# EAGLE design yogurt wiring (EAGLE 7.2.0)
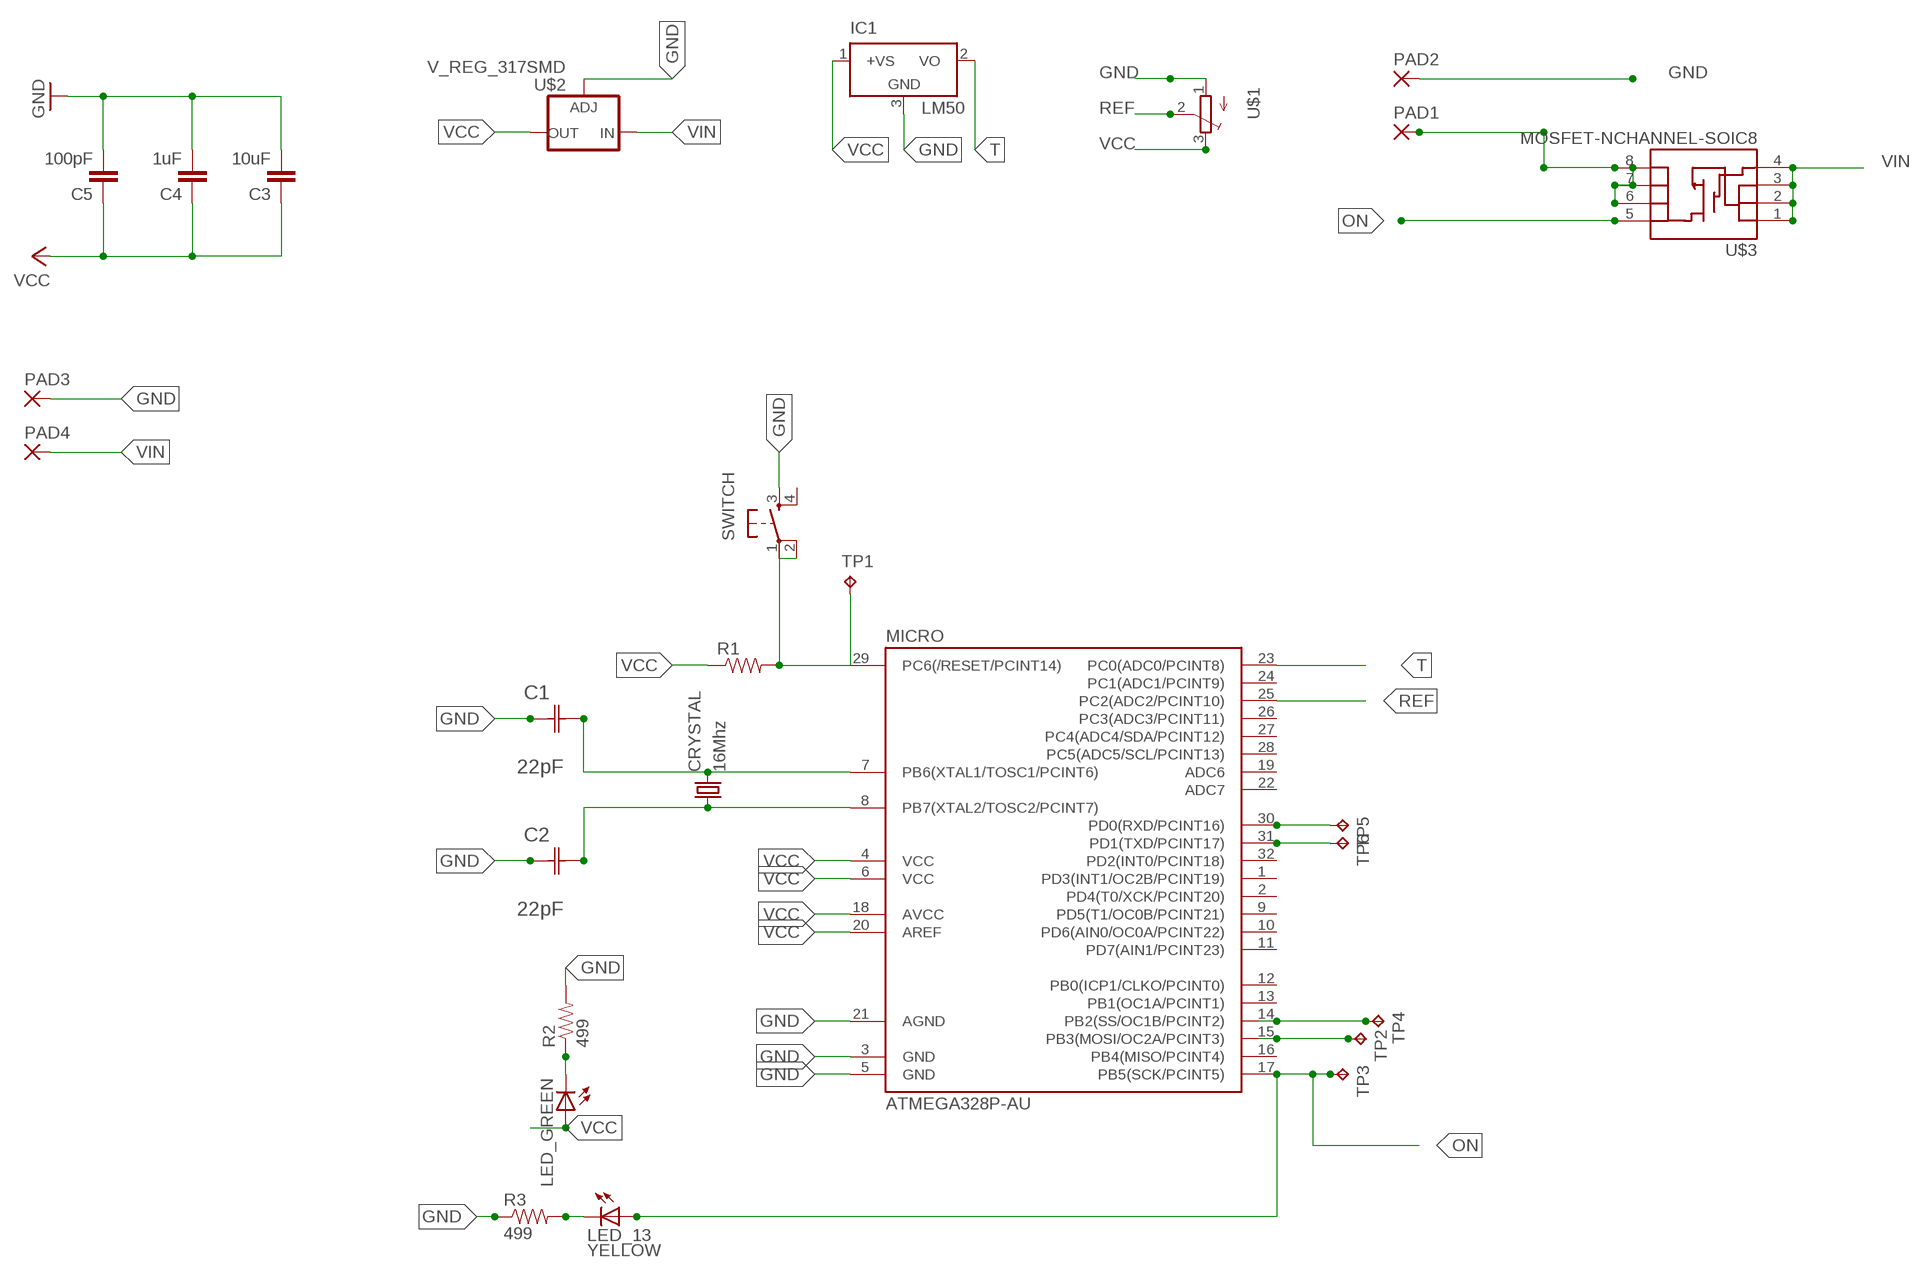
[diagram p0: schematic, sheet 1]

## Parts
C1  22pF  0612ZC225MAT2A  [CAPC3216X178N]
C2  22pF  0612ZC225MAT2A  [CAPC3216X178N]
C3  10uF  CAP1206  [1206]
C4  1uF  CAP1206  [1206]
C5  100pF  CAP1206  [1206]
CRYSTAL  16Mhz  CSM-7X-DU  [CSM-7X-DU]
IC1  LM50  [SOT23]
LED_13  YELLOW  LED1206  [1206]
LED_GREEN  LED1206  [1206]
MICRO  ATMEGA328P-AU  ATMEGA48/88/168-AU  [TQFP32-08]
PAD1  SMD5  [SMD2,54-5,08]
PAD2  SMD5  [SMD2,54-5,08]
PAD3  SMD5  [SMD2,54-5,08]
PAD4  SMD5  [SMD2,54-5,08]
R1  RESISTOR1206  [1206]
R2  499  RESISTOR1206  [1206]
R3  499  RESISTOR1206  [1206]
SWITCH  6MM_SWITCH6MM_SWITCH  [6MM_SWITCH]
TP1  TPPAD1-17Y  [P1-17Y]
TP2  TPPAD1-17Y  [P1-17Y]
TP3  TPPAD1-17Y  [P1-17Y]
TP4  TPPAD1-17Y  [P1-17Y]
TP5  TPPAD1-17Y  [P1-17Y]
TP6  TPPAD1-17Y  [P1-17Y]
U$1  TRIMPOTTC33X  [TC33X]
U$2  V_REG_317SMD  [SOT223]
U$3  MOSFET-NCHANNEL-SOIC8  [SO08]

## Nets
GND: C1.1(C1) C2.1(C1) C3.2 C4.2 C5.2 IC1.3(GND) MICRO.3(GND) MICRO.5(GND) MICRO.21(AGND) PAD2.1(P) PAD3.1(P) R2.2 R3.1 SWITCH.3(S) U$1.1(A) U$2.1(ADJ)
N$2: C1.2(C2) CRYSTAL.2 MICRO.7(PB6(XTAL1/TOSC1/PCINT6))
N$4: MICRO.29(PC6(/RESET/PCINT14)) R1.2 SWITCH.1(P) SWITCH.2(P1) TP1.TP
N$5: MICRO.15(PB3(MOSI/OC2A/PCINT3)) TP2.TP
N$6: MICRO.14(PB2(SS/OC1B/PCINT2)) TP4.TP
N$7: MICRO.31(PD1(TXD/PCINT17)) TP6.TP
N$8: MICRO.30(PD0(RXD/PCINT16)) TP5.TP
N$9: C2.2(C2) CRYSTAL.1 MICRO.8(PB7(XTAL2/TOSC2/PCINT7))
N$26: LED_GREEN.2(C) R2.1
N$27: LED_13.2(C) R3.2
N$35: U$3.6(D) U$3.7(D)
N$36: PAD1.1(P) U$3.8(D)
ON: LED_13.1(A) MICRO.17(PB5(SCK/PCINT5)) TP3.TP U$3.5(D)
REF: MICRO.25(PC2(ADC2/PCINT10)) U$1.2(S)
T: IC1.2(VO) MICRO.23(PC0(ADC0/PCINT8))
VCC: C3.1 C4.1 C5.1 IC1.1(+VS) LED_GREEN.1(A) MICRO.4(VCC) MICRO.6(VCC) MICRO.18(AVCC) MICRO.20(AREF) R1.1 U$1.3(E) U$2.2(OUT)
VIN: PAD4.1(P) U$2.3(IN) U$3.1(S) U$3.2(S) U$3.3(S) U$3.4(G)
Unconnected: MICRO.1(PD3(INT1/OC2B/PCINT19)) MICRO.2(PD4(T0/XCK/PCINT20)) MICRO.9(PD5(T1/OC0B/PCINT21)) MICRO.10(PD6(AIN0/OC0A/PCINT22)) MICRO.11(PD7(AIN1/PCINT23)) MICRO.12(PB0(ICP1/CLKO/PCINT0)) MICRO.13(PB1(OC1A/PCINT1)) MICRO.16(PB4(MISO/PCINT4)) MICRO.19(ADC6) MICRO.22(ADC7) MICRO.24(PC1(ADC1/PCINT9)) MICRO.26(PC3(ADC3/PCINT11)) MICRO.27(PC4(ADC4/SDA/PCINT12)) MICRO.28(PC5(ADC5/SCL/PCINT13)) MICRO.32(PD2(INT0/PCINT18)) SWITCH.4(S1)

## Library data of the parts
C1 C2 = AVX_By_element14_Batch_1:0612ZC225MAT2A: Capacitor 1206; MPN: 0612ZC225MAT2A; OC_FARNELL: -; OC_NEWARK: 12N3209; SUPPLIER: AVX; TOLERANCE: ±20%; VALUE: 2.2µF; VOLTAGERATING: 10V
C3-C5 = 01_SparkFun:CAP: Capacitor
CRYSTAL = 01_FAB_Hello:CSM-7X-DU: SMD CRYSTAL; OC_FARNELL: unknown; OC_NEWARK: unknown
IC1 = linear:LM50: SOT-23 Single-Supply Centigrade Temperature Sensor Vout = (10mV/°C x Temp °C) +5mmmV Source: http://cache.national.com/ds/LM/LM50.pdf
LED_13 LED_GREEN = 01_FAB_Hello:LED
MICRO = atmega8:ATMEGA48/88/168
PAD1-PAD4 = wirepad:SMD5: SMD PAD
R1-R3 = 01_SparkFun:RESISTOR: Resistor
SWITCH = 01_FAB_Hello:6MM_SWITCH: OMRON SWITCH
TP1-TP6 = testpad:TP: Test pad
U$1 = 01_adafruit:TRIMPOT: SMT trimmer potentiometer part number TC33X http://www.ladyada.net/library/eagle
U$2 = 01_SparkFun:V_REG_317: Voltage Regulator Standard LM317 adjustable voltage regulator. AOI (Adjust Output Input). Google 'LM317 Calculator' for easy to use app to get the two resistor values needed. 240/720 for 5V output. 240/390 for 3.3V output. Spark Fun Electronics SKU : COM-00527
U$3 = 01_SparkFun:MOSFET-NCHANNEL-SOIC8: N-Channel MOSFET IRF9410 and NDS8434 are common, SOIC-8 parts.

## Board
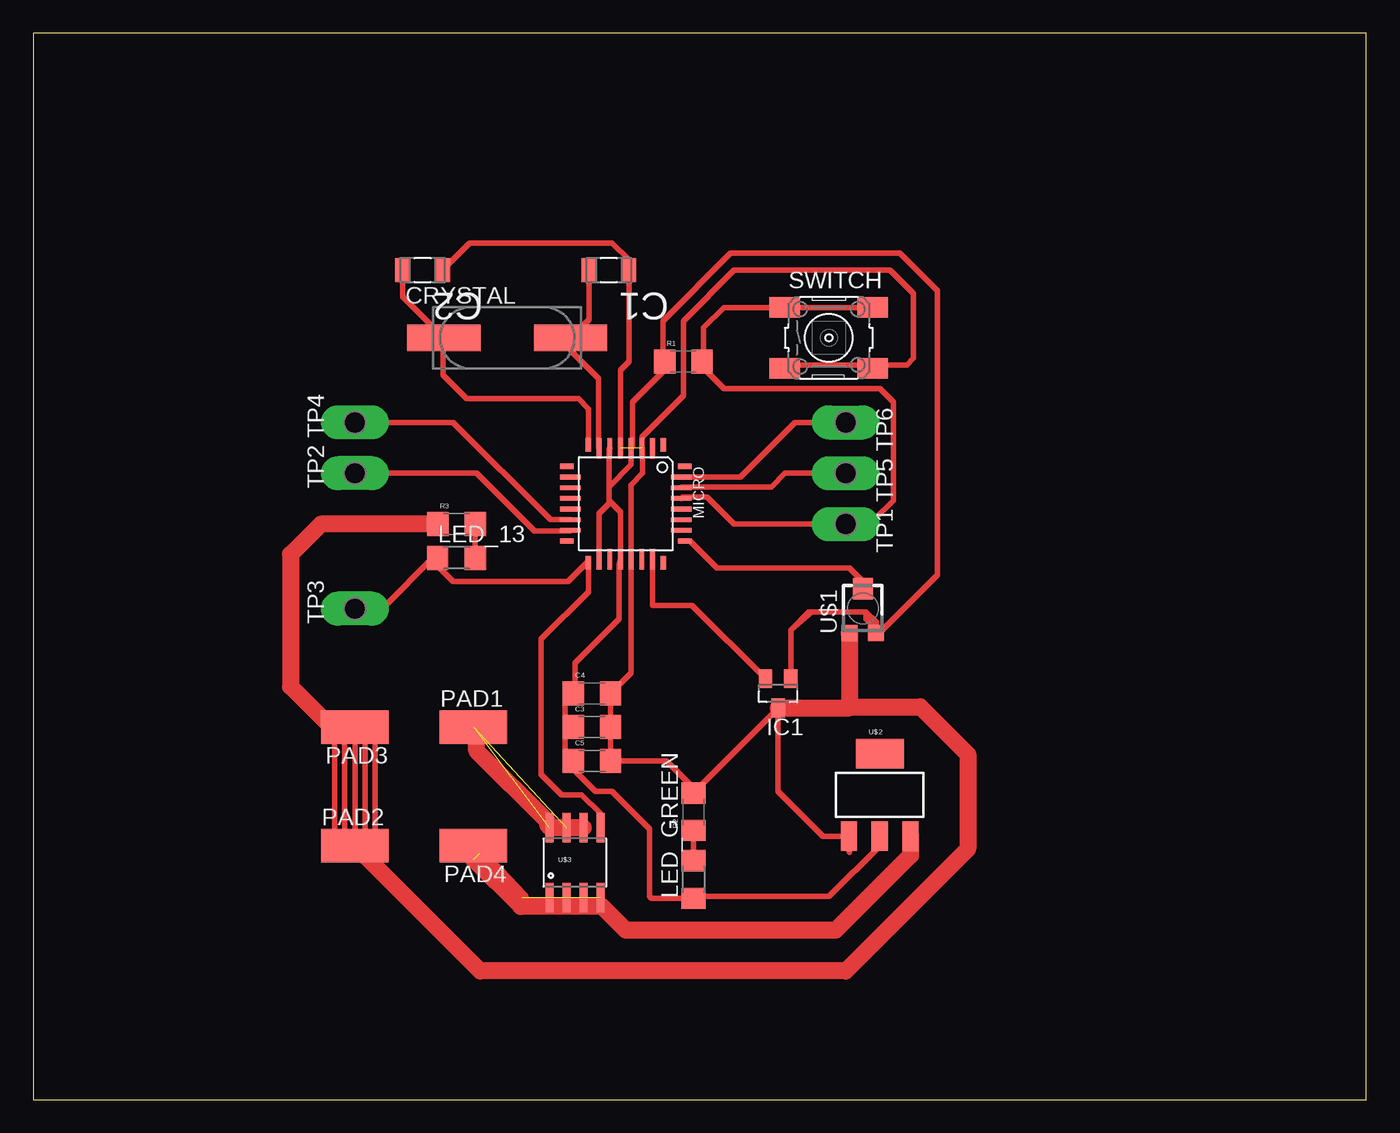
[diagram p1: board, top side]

Size 100 x 80 mm. Coordinates in mm from the lower left corner, seen from the top.
Outline: 0,0 100,0 100,80 0,80 0,0
Copper layers (1*16): Top 0.035mm / dielectric 1.5mm / Bottom 0.035mm
Design rules "default *": minimum track width 16mil, minimum drill 24mil, track to track 12mil, track to pad 12mil, pad to pad 12mil, via to via 12mil, smd to smd 12mil, copper to edge 40mil, drill to drill 8mil, minimum pad ring 10mil, minimum via ring 8mil, stop-mask expansion 4mil, vias tented up to drill 0mil, thermal gap 10mil

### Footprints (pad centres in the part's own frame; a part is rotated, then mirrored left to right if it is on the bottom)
CAPC3216X178N = smd 1.118 x 1.803: 1 -1.499,0; 2 1.499,0
1206 = smd 1.6 x 1.8: 1 -1.4,0; 2 1.4,0
CSM-7X-DU = smd 5.5 x 2: 1 -4.75,0; 2 4.75,0
SOT23 = smd 1 x 1.4: 1 -0.95,-1.1; 2 0.95,-1.1; 3 0,1.1
1206' = smd 1.6 x 1.803: 1 -1.422,0; 2 1.422,0
TQFP32-08 = smd 1.016 x 0.406: 1 -4.42,2.8; 8 -4.42,-2.8; 17 4.42,-2.8; 24 4.42,2.8 | smd 1.524 x 0.356: 2 -4.166,2; 3 -4.166,1.2; 4 -4.166,0.4; 5 -4.166,-0.4; 6 -4.166,-1.2; 7 -4.166,-2; 18 4.166,-2; 19 4.166,-1.2; 20 4.166,-0.4; 21 4.166,0.4; 22 4.166,1.2; 23 4.166,2 | smd 0.406 x 1.016: 9 -2.8,-4.42; 16 2.8,-4.42; 25 2.8,4.42; 32 -2.8,4.42 | smd 0.356 x 1.524: 10 -2,-4.166; 11 -1.2,-4.166; 12 -0.4,-4.166; 13 0.4,-4.166; 14 1.2,-4.166; 15 2,-4.166; 26 2,4.166; 27 1.2,4.166; 28 0.4,4.166; 29 -0.4,4.166; 30 -1.2,4.166; 31 -2,4.166
SMD2,54-5,08 = smd 2.54 x 5.08: 1 0,0
6MM_SWITCH = smd 2.286 x 1.524: 1 -3.302,2.286; 2 3.302,2.286; 3 -3.302,-2.286; 4 3.302,-2.286
P1-17Y = drill 1.702 pad 2.121 long: TP 0,0
TC33X = smd 1.2 x 1.2: 1 -1,-1.825; 3 1,-1.825 | smd 1.5 x 1.6: 2 0,1.5
SOT223 = smd 1.219 x 2.235: 1 -2.311,-3.099; 2 0,-3.099; 3 2.311,-3.099 | smd 3.6 x 2.2: 4 0,3.099
SO08 = smd 0.61 x 2.21: 1 -1.905,-2.616; 2 -0.635,-2.616; 3 0.635,-2.616; 4 1.905,-2.616; 5 1.905,2.616; 6 0.635,2.616; 7 -0.635,2.616; 8 -1.905,2.616

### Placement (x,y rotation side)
C1  43.18,62.23 180 top
C2  29.21,62.23 180 top
C3  41.91,27.94 0 top
C4  41.91,30.48 0 top
C5  41.91,25.4 0 top
CRYSTAL  35.56,57.15 0 top
IC1  55.88,30.48 180 top
LED_13  YELLOW  [1206']  31.75,40.64 0 top
LED_GREEN  [1206']  49.53,16.51 90 top
MICRO  44.45,44.7 270 top
PAD1  33.02,27.94 270 top
PAD2  24.13,19.05 270 top
PAD3  24.13,27.94 90 top
PAD4  33.02,19.05 90 top
R1  48.77,55.37 0 top
R2  49.53,21.59 90 top
R3  31.75,43.18 0 top
SWITCH  59.69,57.15 0 top
TP1  60.96,43.18 270 top
TP2  24.13,46.99 90 top
TP3  24.13,36.83 90 top
TP4  24.13,50.8 90 top
TP5  60.96,46.99 270 top
TP6  60.96,50.8 270 top
U$1  62.23,36.83 0 top
U$2  63.5,22.86 0 top
U$3  40.64,17.78 0 top

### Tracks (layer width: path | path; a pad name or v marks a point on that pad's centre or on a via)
GND  (1 unrouted)
  Top 0.406: PAD3.1 PAD2.1 | U$2.1 59.23,19.76 55.88,23.11 IC1.3 55.88,29.34 R2.2 49.53,23.37 47.5,25.4 C5.2 C3.2 C4.2 44.85,32.02 MICRO.21 44.85,46.12 45.72,46.99 45.72,48.8 MICRO.3 45.65,49.71 48.77,52.83 48.77,58.42 52.58,62.23 64.26,62.23 66.04,60.45 66.04,55.63 65.53,55.12 56.64,55.12 SWITCH.3 | MICRO.5 44.05,54.72 44.7,55.37 44.7,62.2 C1.1 44.68,63.02 43.43,64.26 32.74,64.26 C2.1
  Top 1.27: U$1.1 61.23,29.46 | 61.23,29.46 66.55,29.46 70.1,25.91 70.1,18.8 60.96,9.65 33.53,9.65 PAD2.1 | R3.1 21.59,43.18 19.3,40.89 19.3,30.99 22.35,27.94 PAD3.1 | IC1.3 61.15,29.38 61.23,29.46
N$1
  Top 0.406: 60.96,19.56 61.21,18.54
N$2
  Top 0.406: C1.2 41.68,58.52 CRYSTAL.2 40.31,56.21 42.42,54.1 42.42,48.9 MICRO.7
N$4
  Top 0.406: MICRO.29 48.72,45.21 50.55,45.21 52.58,43.18 TP1.TP 61.21,43.43 62.99,43.43 64.52,44.96 64.52,52.32 63.5,53.34 51.82,53.34 50.17,54.99 R1.2 50.29,55.5 50.29,57.91 51.82,59.44 SWITCH.1 SWITCH.2
N$5
  Top 0.406: TP2.TP 33.27,46.99 37.59,42.67 40.25,42.67 MICRO.15
N$6
  Top 0.406: MICRO.14 38.79,43.5 31.5,50.8 24.89,50.8 24.64,50.55 24.38,50.55 TP4.TP
N$7
  Top 0.406: MICRO.31 53.05,46.7 57.15,50.8 TP6.TP
N$8
  Top 0.406: TP5.TP 56.39,46.99 55.37,45.97 48.69,45.97 MICRO.30
N$9
  Top 0.406: MICRO.8 41.65,51.82 40.89,52.58 32.51,52.58 30.73,54.36 30.73,57.07 CRYSTAL.1 27.71,60.25 C2.2
N$10
  Top 0.406: 22.61,27.69 22.61,19.3 23.37,20.07 23.37,27.43 23.62,27.18 25.15,27.18 24.89,26.92 24.89,19.56 25.15,19.81 25.91,19.81 25.65,20.07 25.65,27.69
N$26
  Top 0.406: LED_GREEN.2 R2.1
N$27
  Top 0.406: R3.2 33.15,40.66 LED_13.2
N$35  (1 unrouted)
  Top 1.27: U$3.6 38.79,20.4 38.61,20.57 38.61,20.83 33.27,26.16 33.27,27.69 33.02,27.94
N$36  (1 unrouted)
ON
  Top 0.406: LED_13.1 29.97,40.64 29.84,40.51 | 29.84,40.51 26.42,37.08 TP3.TP | U$3.5 42.55,21.46 41.15,22.86 39.62,22.86 38.1,24.38 38.1,34.54 41.66,38.1 MICRO.17 41.55,40.28 40.13,38.86 31.5,38.86 29.84,40.51
REF
  Top 0.406: U$1.2 62.23,38.86 61.21,39.88 51.31,39.88 49.28,41.91 MICRO.25
T
  Top 0.406: IC1.2 49.43,37.08 46.48,37.08 46.45,37.12 MICRO.23
VCC
  Top 0.406: U$2.2 63.5,19.05 59.69,15.24 49.68,15.24 LED_GREEN.1 46.38,15.09 46.23,15.24 46.23,20.32 43.43,23.11 42.16,23.11 40.26,25.02 | 39.88,27.94 39.88,29.85 C4.1 40.64,30.61 40.64,32.77 43.94,36.07 43.94,40.14 MICRO.20 44.05,44.09 43.31,44.83 | 39.88,27.94 39.88,25.4 40.26,25.02 | C5.1 40.26,25.15 40.26,25.02 | C3.1 39.88,27.94 | 43.31,44.83 43.18,44.96 43.18,45.97 | 43.18,45.97 43.18,48.8 MICRO.6 | MICRO.18 42.45,43.97 43.31,44.83 | 43.18,45.97 44.85,47.64 MICRO.4 44.96,48.98 44.96,52.32 47.37,54.73 R1.1 47.24,55.5 47.24,58.42 52.32,63.5 65.02,63.5 67.82,60.71 67.82,39.37 63.5,35.05 62.48,36.07 62.48,36.58 | IC1.1 56.83,35.24 | 56.83,35.24 58.42,36.58 | 58.42,36.58 62.48,36.58 | 62.48,36.58 63.25,35.81 63.25,35.02 U$1.3 | 56.83,35.24 58.17,36.58 58.42,36.58
VIN  (5 unrouted)
  Top 1.016: PAD4.1 36.65,15.16
  Top 1.27: U$2.3 65.81,18.31 60.2,12.7 44.45,12.7 42.67,14.48 36.58,14.48 33.02,18.03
